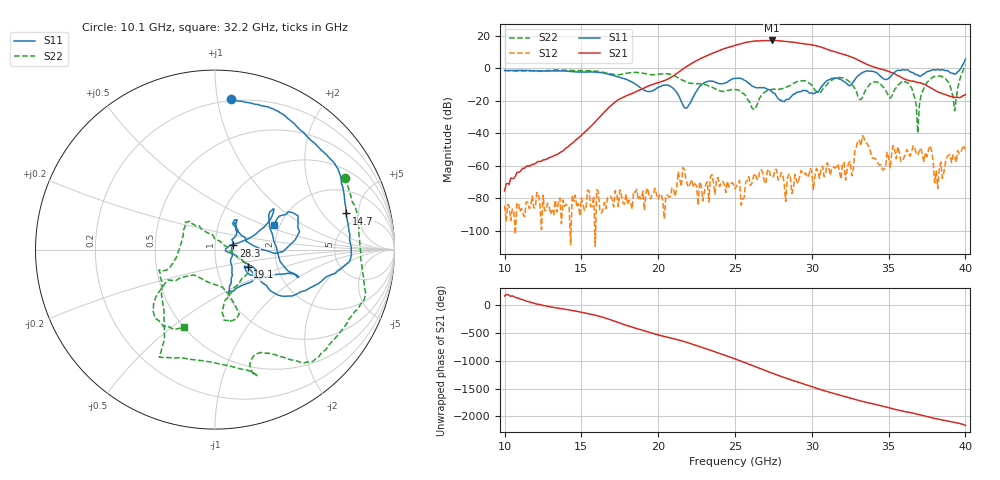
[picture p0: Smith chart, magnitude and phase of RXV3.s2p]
!Keysight Technologies,M9808A,MY58100618,A.14.70.03
!Date: Monday, February 27, 2023 13:25:38
!Correction: S11(Cdelta 2-Port  )
!S21(Cdelta 2-Port  )
!S12(Cdelta 2-Port  )
!S22(Cdelta 2-Port  )
!S2P File: Measurements: S11, S21, S12, S22:
# Hz S  RI  R 50
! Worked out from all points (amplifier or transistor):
!   301 points, 10 GHz to 40 GHz, reference 50 ohm
!   highest |S21| = 17.0 dB at 27.4 GHz (marker M1)
!   |S21| within 3 dB of that: 25.01 GHz to 30.17 GHz (5.159 GHz wide, 18.7 % of centre)
!   unconditionally stable (mu >= 1): start of sweep to 39.72 GHz
!   at 15 GHz: K = 77197.07, MAG = -32.6 dB, |S12| = -79.8 dB
!   at 25 GHz: K = 380.63, MAG = 15.3 dB, |S12| = -74.3 dB
!   at 40 GHz: K = 1526.66, MSG = 17.0 dB, |S12| = -50.2 dB
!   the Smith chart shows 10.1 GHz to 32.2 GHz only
!   S11 on the Smith chart (normalised r, x): 10.1 GHz: 0.19, +1.10; 14.7 GHz: 3.75, +3.54; 19.1 GHz: 1.41, -0.29; 28.3 GHz: 1.23, +0.06; 32.2 GHz: 1.86, +0.59
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1e10  0.0678 0.84  -0.000164 3.19e-05  -1.93e-05 5.62e-05  0.7136 0.4319
1.01e10  0.0911 0.8375  -0.000267 -5.73e-05  -1.91e-05 -5.43e-07  0.723 0.4013
1.47e10  0.7296 0.2015  -0.00196 -0.00625  9.45e-07 -5.27e-05  0.6831 -0.4777
1.5e10  0.7453 0.1093  -0.00498 -0.00707  -0.000101 1.35e-05  0.6313 -0.5347
1.91e10  0.182 -0.0986  -0.0404 -0.2433  -3.23e-05 -2.84e-05  0.1515 -0.6671
2e10  0.2101 -0.1418  -0.3527 -0.0425  7.49e-05 -5.23e-05  -0.227 -0.6044
2.27e10  0.2501 0.1075  1.723 -0.7969  0.000129 0.00029  -0.307 -0.116
2.37e10  0.3044 0.2089  -1.438 -2.699  6.95e-05 -0.000114  -0.2248 -0.0591
2.44e10  0.3509 -0.0261  -4.049 0.4323  -0.000128 7.9e-05  -0.1755 0.0831
2.5e10  0.4571 -0.1523  -1.972 4.574  0.000155 -0.000114  -0.1591 0.1514
2.56e10  0.4033 -0.1325  3.618 4.716  -6.72e-05 8.21e-05  -0.0876 0.1319
2.62e10  0.2035 -0.1793  6.513 -1.614  -0.000468 3.83e-05  0.0289 0.0462
2.68e10  0.0804 -0.2328  1.332 -6.819  -0.000624 5.49e-05  0.1456 -0.0576
2.74e10  0.0901 -0.163  -5.485 -4.433  0.000395 0.000194  0.1899 -0.1111
2.78e10  0.0894 -0.0771  -6.92 0.3032  0.000359 -4.5e-05  0.1514 -0.1585
2.83e10  0.1018 0.0234  -4.111 5.125  -9.23e-06 7.86e-05  0.0923 -0.2398
2.92e10  0.1122 0.1488  4.093 4.128  -0.00041 -0.000163  0.0584 -0.3945
3e10  0.1255 0.1136  4.636 -2.314  -0.00065 -4.38e-05  0.097 -0.2837
3.11e10  0.433 0.0404  -1.98 -3.038  -0.000696 0.000677  -0.294 -0.211
3.22e10  0.3287 0.1382  -2.202 1.209  -0.000239 0.000268  -0.1712 -0.4324
3.5e10  0.4578 -0.1471  0.5547 -0.561  7.87e-05 -0.00184  0.0107 -0.1391
4e10  1.042 -1.564  0.1527 -0.0157  -0.00276 0.00137  0.5819 -1.11
